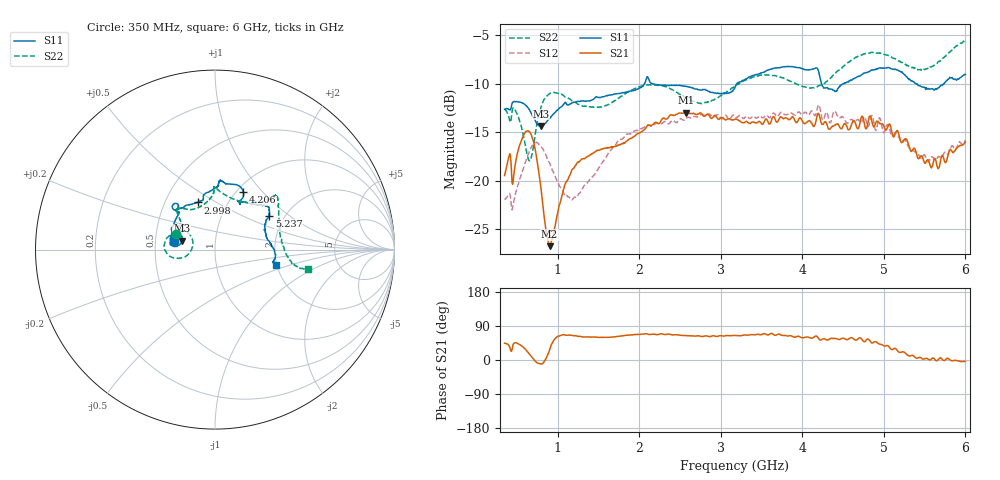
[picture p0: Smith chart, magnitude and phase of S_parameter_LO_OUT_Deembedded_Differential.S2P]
!Agilent Technologies,E5071B,MY42403504,A.06.51
!Date: Mon Mar 10 13:20:12 2014
!Data & Calibration Information:
!Freq	S33:SOLT2(ON)	S43:SOLT2(ON)	S34:SOLT2(ON)	S44:SOLT2(ON)
# Hz S dB R 50
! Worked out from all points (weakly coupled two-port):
!   801 points, 350 MHz to 6 GHz, reference 50 ohm
!   highest |S21| = -13.00 dB at 2.575 GHz (marker M1); lowest = -26.7 dB at 900.9 MHz (marker M2)
!   lowest |S11| = -14.4 dB at 794.9 MHz (marker M3), VSWR 1.47, Z = 34.2 + j3.47 ohm
!   |S11| at or under -10 dB: start of sweep to 2.066 GHz; 2.158 GHz to 3.201 GHz (1.042 GHz wide, 38.9 % of centre); 5.393 GHz to 5.739 GHz (346.9 MHz wide, 6.23 % of centre)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
!   |S22| runs from -18.0 to -5.6 dB; largest |S21 - S12| = 0.1
!   S11 on the Smith chart (normalised r, x): 350 MHz: 0.63, +0.06; 2.998 GHz: 0.72, +0.41; 4.206 GHz: 1.08, +0.79; 5.237 GHz: 1.67, +0.72; 6 GHz: 1.98, -0.39
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3.5e8  -12.65 168.3  -19.47 44.2  -21.93 24.8  -12.64 158.2
4.9125e8  -11.85 163.4  -17.78 45.2  -21.06 47.0  -12.94 152.3
6.395625e8  -12.52 155.7  -14.86 19.5  -17.29 47.7  -17.76 161.8
7.101875e8  -13.56 156.3  -16.13 0.9  -16.27 38.8  -16.10 -168.8
7.949375e8  -14.36 165.2  -20.68 -10.3  -16.49 26.5  -12.47 -169.0
9.00875e8  -13.61 174.2  -26.74 26.6  -18.18 19.1  -11.03 179.8
1.105688e9  -12.05 170.5  -20.09 65.4  -21.50 33.3  -11.44 164.4
1.296375e9  -11.79 163.7  -17.76 61.4  -20.97 57.8  -12.27 154.7
1.748375e9  -11.03 137.5  -16.30 62.6  -15.86 70.4  -11.51 138.4
2.235688e9  -10.14 131.4  -14.13 67.4  -14.12 64.8  -10.17 132.4
2.574688e9  -10.29 132.3  -13.00 64.4  -13.62 67.7  -11.54 122.8
2.998438e9  -11.05 110.2  -13.56 64.0  -13.57 66.9  -11.27 98.1
3.175e9  -10.39 102.5  -13.67 64.8  -13.38 69.6  -10.24 92.5
3.577562e9  -8.61 86.7  -13.89 66.0  -13.36 70.9  -9.10 90.9
4.121375e9  -8.52 77.2  -14.18 57.6  -12.84 60.1  -10.44 68.1
4.206125e9  -8.97 63.7  -13.21 55.1  -12.23 55.9  -10.24 60.8
4.396812e9  -10.80 61.1  -14.28 57.0  -12.83 55.8  -9.02 48.3
4.749938e9  -8.97 44.4  -13.64 49.4  -13.52 52.2  -6.97 42.3
5.060688e9  -8.37 37.7  -14.21 35.7  -14.42 29.0  -7.14 36.4
5.23725e9  -8.96 31.8  -15.99 21.2  -15.88 18.3  -7.93 28.1
5.668062e9  -10.44 10.1  -18.77 1.2  -17.50 2.2  -7.75 -6.2
6e9  -9.07 -14.3  -16.02 -3.7  -15.81 -1.1  -5.57 -11.7
